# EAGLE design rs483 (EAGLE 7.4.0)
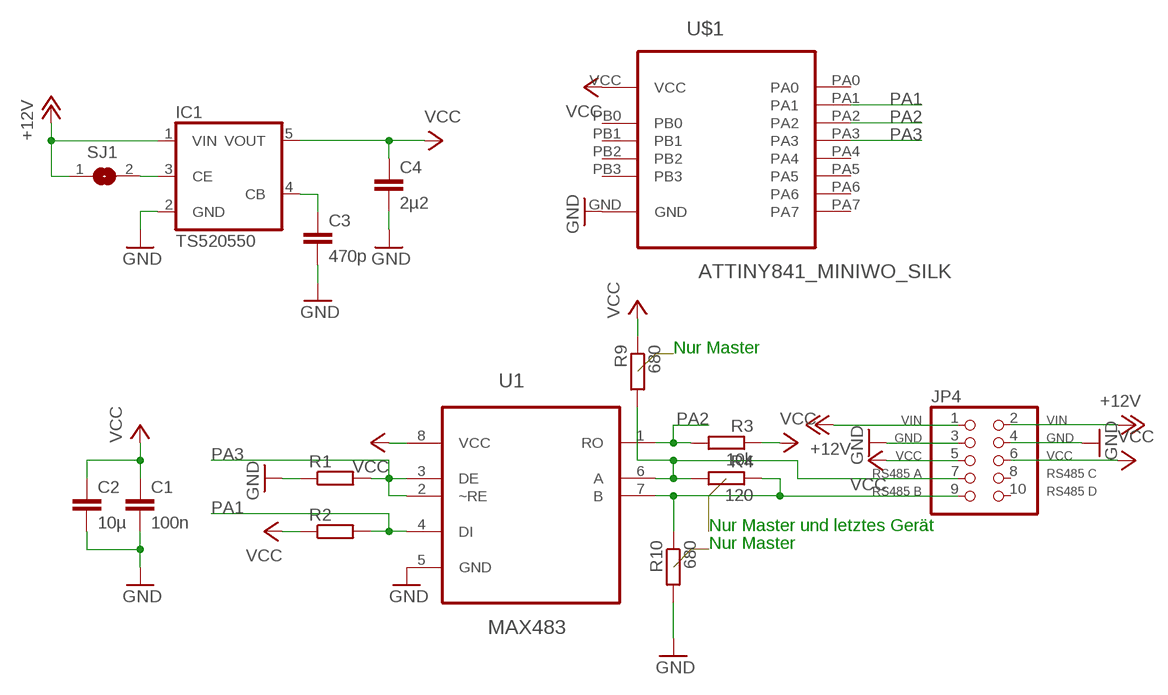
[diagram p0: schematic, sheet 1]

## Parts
C1  100n  C-EUC0805  [C0805]
C2  10µ  C-EUC0805  [C0805]
C3  470p  C-EUC0805  [C0805]
C4  2µ2  C-EUC0805  [C0805]
IC1  TS520550  [SOT25]
JP4  PINHD-2X5_RS485_2.54  [2X05]
R1  R-EU_M0805  [M0805]
R2  R-EU_M0805  [M0805]
R3  10k  R-EU_M0805  [M0805]
R4  120  R-EU_M0805  [M0805]
R9  680  R-EU_M0805  [M0805]
R10  680  R-EU_M0805  [M0805]
SJ1  SJ  [SJ]
U1  MAX483  MAX485ECSA+  [SOIC127P600X175-8N]
U$1  ATTINY841_MINIWO_SILK  [ATTINY841_BOARD_WO_SILK]

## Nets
+12V: IC1.1(VIN) JP4.1 JP4.2 SJ1.1
GND: C1.2 C2.2 C3.2 C4.2 IC1.2(GND) JP4.3 JP4.4 R1.1 R10.2 U1.5(GND) U$1.GND
N$5: C3.1 IC1.4(CB)
N$8: JP4.9 R4.1 R10.1 U1.7(B)
N$11: JP4.7 R4.2 R9.2 U1.6(A)
N$12: IC1.3(CE) SJ1.2
PA1: R2.2 U1.4(DI) U$1.PA1
PA2: R3.2 U1.1(RO) U$1.PA2
PA3: R1.2 U1.2(~RE) U1.3(DE) U$1.PA3
VCC: C1.1 C2.1 C4.1 IC1.5(VOUT) JP4.5 JP4.6 R2.1 R3.1 R9.1 U1.8(VCC) U$1.VCC
Unconnected: JP4.8 JP4.10 U$1.PA0 U$1.PA4 U$1.PA5 U$1.PA6 U$1.PA7 U$1.PB0 U$1.PB1 U$1.PB2 U$1.PB3

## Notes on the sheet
- Nur Master
- Nur Master und letztes Gerät
- Nur Master

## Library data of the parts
C1-C4 = rcl:C-EU: CAPACITOR, European symbol
IC1 = v-reg:TS5205: 150mA Low Noise LDO Voltage Regulator with Enable TSC [Taiwan Semiconductor Company, Ltd] Source: http://www.taiwansemi.com .. 5205_0409c.pdf
JP4 = pinhead:PINHD-2X5_RS485: PIN HEADER
R1-R4 R9 R10 = rcl:R-EU_: RESISTOR, European symbol
SJ1 = jumper:SJ: SMD solder JUMPER
U1 = Maxim_By_element14_Batch_1:MAX485ECSA+: ±15kV ESD-Protected, Slew-Rate-Limited, Low-Power, RS-485/RS-422 Transceivers; MPN: MAX485ECSA+; OC_FARNELL: 9724524; OC_NEWARK: 68K4797; PACKAGE: SOIC-8; SUPPLIER: Maxim
U$1 = _ssr:ATTINY841_MINI

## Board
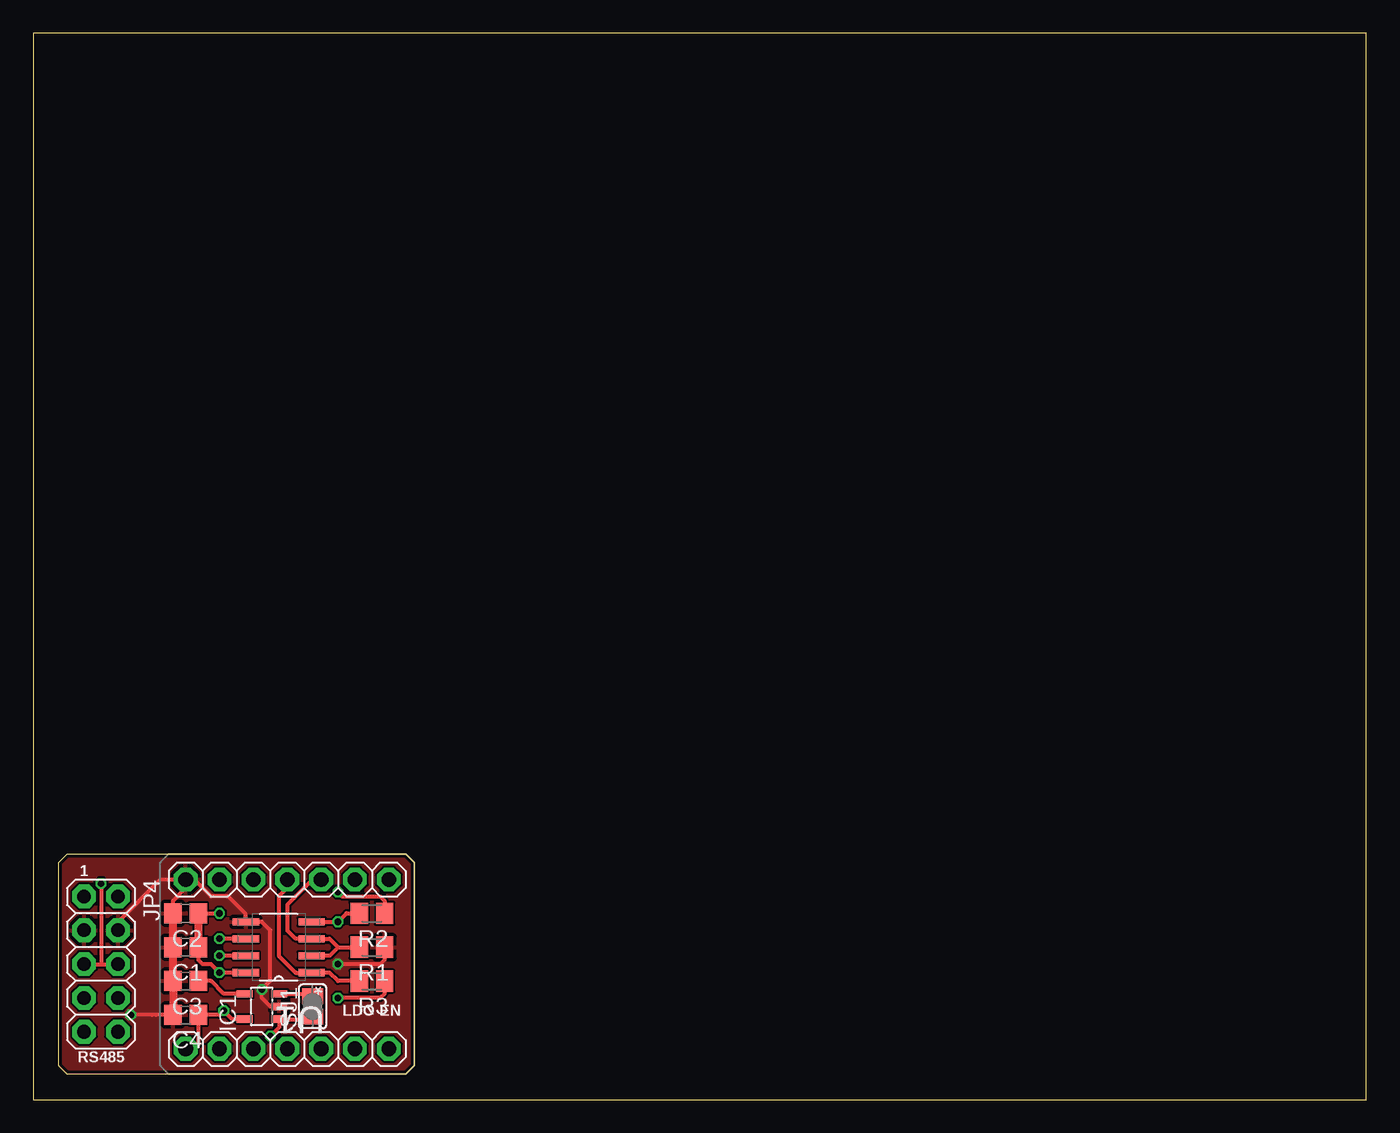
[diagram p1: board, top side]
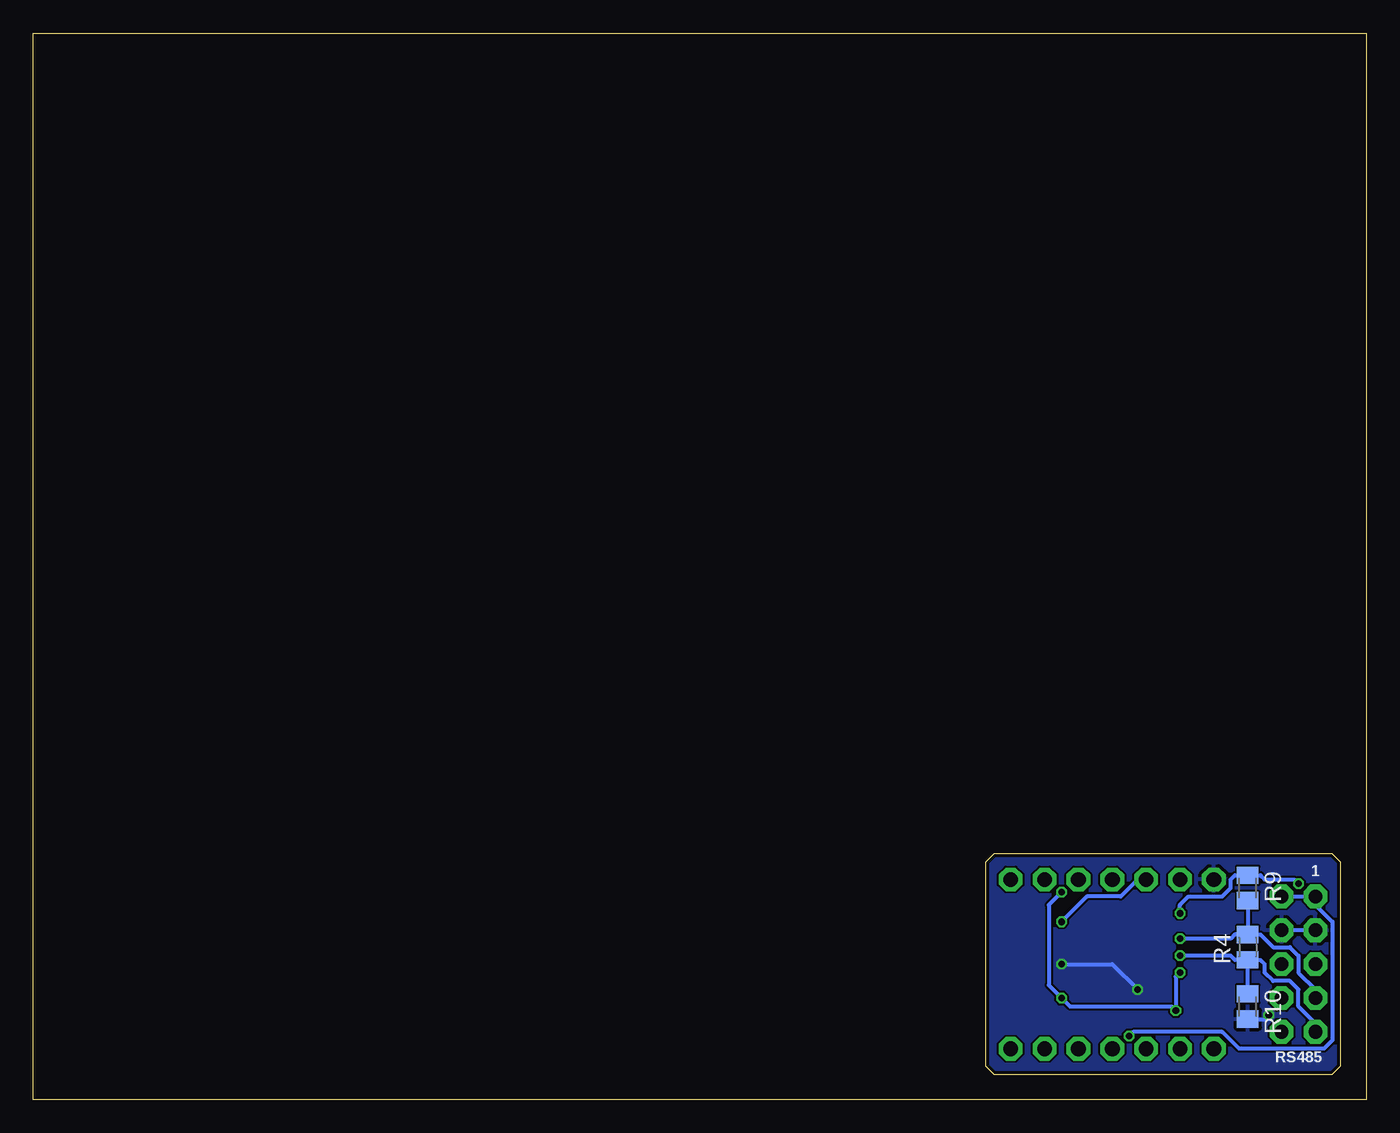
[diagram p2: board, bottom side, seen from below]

Size 100 x 80 mm. Coordinates in mm from the lower left corner, seen from the top.
Outline: 0,0 100,0 100,80 0,80 0,0
Outline: 1.91,17.78 2.54,18.41 27.94,18.41 28.57,17.78 28.57,2.54 27.94,1.91 2.54,1.91 1.91,2.54 1.91,17.78
Copper layers (1*16): Top 0.035mm / dielectric 1.5mm / Bottom 0.035mm
Design rules "Elecrow_2-layer_eagle_rule": minimum track width 6mil, minimum drill 12mil, track to track 6mil, track to pad 6mil, pad to pad 6mil, via to via 6mil, smd to smd 0mil, copper to edge 10mil, drill to drill 10mil, minimum pad ring 10mil, minimum via ring 6mil, stop-mask expansion 2mil, vias tented up to drill 100mil, thermal gap 10mil

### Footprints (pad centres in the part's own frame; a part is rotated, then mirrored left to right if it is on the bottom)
C0805 = smd 1.3 x 1.5: 1 -0.95,0; 2 0.95,0
SOT25 = smd 0.55 x 1.2: 1 -0.95,-1.3; 2 0,-1.3; 3 0.95,-1.3; 4 0.95,1.3; 5 -0.95,1.3
2X05 = drill 1.016 pad 1.778 octagon: 1 -5.08,-1.27; 2 -5.08,1.27; 3 -2.54,-1.27; 4 -2.54,1.27; 5 0,-1.27; 6 0,1.27; 7 2.54,-1.27; 8 2.54,1.27; 9 5.08,-1.27; 10 5.08,1.27
M0805 = smd 1.3 x 1.6: 1 -0.95,0; 2 0.95,0
SJ = smd 1.168 x 1.6: 1 -0.762,0; 2 0.762,0
SOIC127P600X175-8N = smd 1.981 x 0.533: 1 -2.464,1.905; 2 -2.464,0.635; 3 -2.464,-0.635; 4 -2.464,-1.905; 5 2.464,-1.905; 6 2.464,-0.635; 7 2.464,0.635; 8 2.464,1.905
ATTINY841_BOARD_WO_SILK = drill 1.1 pad 1.778 octagon: GND 2.54,15.24; PA0 5.08,15.24; PA1 7.62,15.24; PA2 10.16,15.24; PA3 12.7,15.24; PA4 15.24,15.24; PA5 17.78,15.24; PA6 17.78,2.54; PA7 15.24,2.54; PB0 5.08,2.54; PB1 7.62,2.54; PB2 10.16,2.54; PB3 12.7,2.54; VCC 2.54,2.54

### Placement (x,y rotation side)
C1  11.43,11.43 180 top
C2  11.43,13.97 180 top
C3  11.43,8.89 180 top
C4  11.43,6.35 180 top
IC1  17.14,6.99 90 top
JP4  5.08,10.16 270 top
R1  25.4,11.43 180 top
R2  25.4,13.97 180 top
R3  25.4,8.89 180 top
R4  8.89,11.43 90 bottom
R9  8.89,15.88 270 bottom
R10  8.89,6.99 270 bottom
SJ1  20.95,6.99 90 top
U1  18.41,11.43 180 top
U$1  8.89,1.27 0 top

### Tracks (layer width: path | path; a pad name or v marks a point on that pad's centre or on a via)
+12V  (via drill 0.5)
  Top 0.305: SJ1.1 20.77,6.04 IC1.1 18.45,5.43 v17.78,4.76
  Bottom 0.305: JP4.2 JP4.1 3.81,14.61 2.54,13.34 2.54,4.45 3.17,3.81 9.53,3.81 10.79,5.08 17.46,5.08 v17.78,4.76
GND  (via drill 0.5)
  Top 0.305: R1.1 26.35,10.47 26.04,10.16 v22.86,10.16 | IC1.2 17.78,6.99 17.14,7.62 v17.14,8.26 17.78,8.89 17.78,12.7 17.14,13.34 U1.5 15.88,13.41 15.88,13.97 14.61,15.24 13.34,15.24 12.06,16.51 U$1.GND | U$1.GND 9.53,16.51 6.35,13.34 JP4.4 | C4.2 9.21,6.35 8.89,6.35 7.62,6.35 v7.3,6.35 | C2.2 10.48,14.93 11.43,15.88 U$1.GND
  Top 0.61: C2.2 C1.2 C3.2 C4.2
  Bottom 0.305: JP4.3 JP4.4 | v22.86,10.16 19.05,10.16 v17.14,8.26 | R10.2 7.62,6.04 v7.3,6.35
  pour Bottom: 0.64,19.68 29.84,19.68 29.84,0.64 0.64,0.64
  pour Top: 0.64,19.68 29.84,19.68 29.84,0.64 0.64,0.64
N$5
  Top 0.305: IC1.4 14.29,7.93 13.34,8.89 C3.1
N$8  (via drill 0.5)
  Top 0.305: U1.7 v13.97,10.79
  Bottom 0.305: R10.1 R4.1 | R4.1 9.85,10.48 10.16,10.79 v13.97,10.79 | JP4.9 3.81,5.71 5.08,6.99 5.08,8.26 5.71,8.89 6.99,8.89 7.62,9.53 7.62,10.16 7.94,10.48 R4.1
N$11  (via drill 0.5)
  Top 0.305: U1.6 v13.97,12.06
  Bottom 0.305: R9.2 R4.2 | R4.2 9.85,12.38 10.16,12.06 v13.97,12.06 | R4.2 7.93,12.38 6.99,11.43 5.71,11.43 5.08,10.79 5.08,9.53 3.81,8.26 JP4.7
N$12
  Top 0.305: IC1.3 20.77,7.93 SJ1.2
PA1  (via drill 0.5)
  Top 0.305: 20.95,13.41 U1.4 v22.86,13.34 23.5,13.97 R2.2
  Bottom 0.305: U$1.PA1 17.14,16.51 18.41,15.24 20.95,15.24 v22.86,13.34
PA2
  Top 0.305: U$1.PA2 19.05,15.88 18.41,15.24 18.41,10.79 19.68,9.53 U1.1 22.23,9.53 22.86,8.89 R3.2
PA3
  Top 0.305: U$1.PA3 20.95,16.51 19.05,14.61 19.05,12.7 19.68,12.06 U1.3 22.23,12.06 22.86,11.43 | 22.86,11.43 22.23,10.79 U1.2 | 22.86,11.43 R1.2
VCC  (via drill 0.5)
  Top 0.305: IC1.5 14.92,6.04 v14.29,6.67 13.97,6.35 C4.1 12.38,4.12 12.06,3.81 U$1.VCC | C1.1 12.38,10.48 12.7,10.16 13.34,10.16 v13.97,9.53 U1.8 | v5.08,16.19 5.08,10.16 | JP4.5 5.08,10.16 | 5.08,10.16 JP4.6 | 12.7,14.29 C2.1 v13.97,13.97 | v22.86,15.56 23.18,15.24 26.04,15.24 26.35,14.92 R2.1 | R3.1 26.35,7.93 26.04,7.62 v22.86,7.62
  Top 0.61: C2.1 C1.1
  Bottom 0.305: v13.97,9.53 14.29,9.21 v14.29,6.67 14.61,6.99 22.23,6.99 v22.86,7.62 23.81,8.57 23.81,14.61 v22.86,15.56 | R9.1 7.94,16.83 7.62,16.51 5.4,16.51 v5.08,16.19 | R9.1 8.89,16.51 | v13.97,13.97 13.97,14.61 13.34,15.24 10.79,15.24 10.16,15.88 10.16,16.51 9.84,16.83 R9.1

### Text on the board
tPlace: 1 | LDO EN | RS485
bPlace: 1 | RS485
